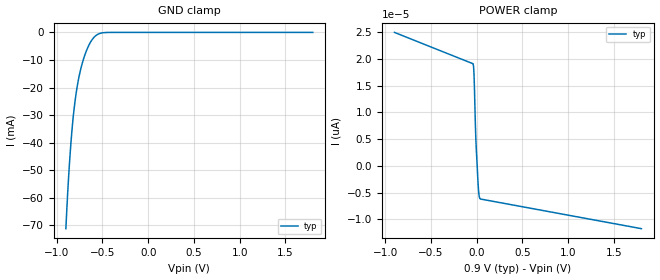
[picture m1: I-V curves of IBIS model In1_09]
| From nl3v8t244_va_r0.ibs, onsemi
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|//////////////////////////////////////////////////////////////////////////////
|//////////////////////////////////////////////////////////////////////////////
[Model]  In1_09
Model_type Input
Vinh =  0.81
Vinl =  0.09
|  variable   typ   min   max
C_comp   6.2pF   6.2pF   6.2pF
|//////////////////////////////////////////////////////////////////////////////
[Temperature Range]   25   125   -40
|//////////////////////////////////////////////////////////////////////////////
[Voltage Range]   0.90V   NA   NA
|//////////////////////////////////////////////////////////////////////////////
[POWER Clamp Reference] 0.90V   NA   NA
|//////////////////////////////////////////////////////////////////////////////
[GND Clamp Reference]   0V   NA   NA
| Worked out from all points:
|   GND clamp passes 1 mA (typ) near -0.57 V on its own axis
|//////////////////////////////////////////////////////////////////////////////
[GND Clamp]
|   Voltage   I(typ)   I(min)   I(max)
-900mV    -71.17mA   NA         NA
-880mV    -58.1mA    NA         NA
-870mV    -52.38mA   NA         NA
-840mV    -38.09mA   NA         NA
-810mV    -27.71mA   NA         NA
-780mV    -20.38mA   NA         NA
-740mV    -13.65mA   NA         NA
-690mV    -7.952mA   NA         NA
-630mV    -3.503mA   NA         NA
-570mV    -1.104mA   NA         NA
-430mV    -13.71uA   NA         NA
1.8V      -3.229pA   NA         NA
|//////////////////////////////////////////////////////////////////////////////
[POWER Clamp]
|   Voltage   I(typ)   I(min)   I(max)
-900mV    24.95pA    NA         NA
-40mV     19.09pA    NA         NA
-35mV     18.58pA    NA         NA
-30mV     17.13pA    NA         NA
-25mV     14.37pA    NA         NA
-15mV     7.634pA    NA         NA
-10mV     5.037pA    NA         NA
-5mV      3.078pA    NA         NA
15mV      -3.465pA   NA         NA
25mV      -5.478pA   NA         NA
40mV      -6.189pA   NA         NA
1.8V      -11.73pA   NA         NA
